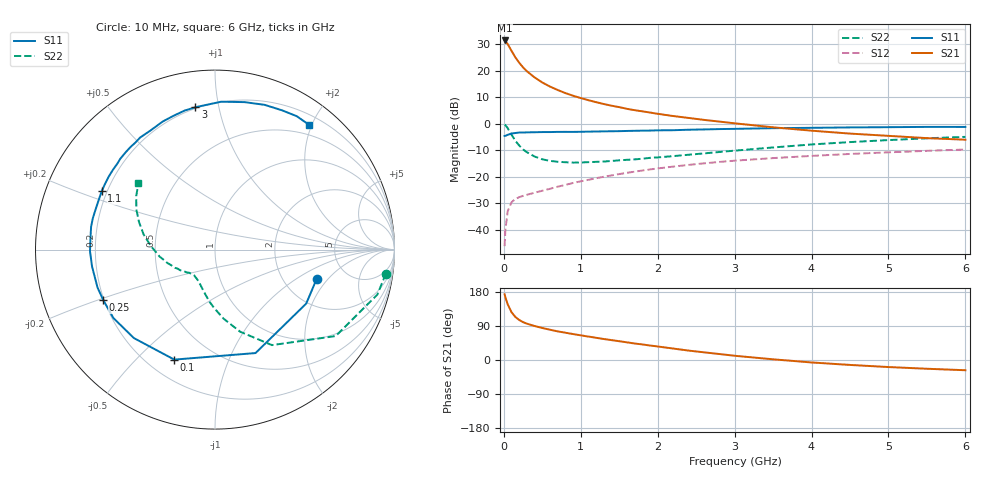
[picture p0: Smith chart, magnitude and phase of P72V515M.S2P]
! SIEMENS Small Signal Semiconductors
! BFP196
! Si NPN RF Bipolar Junction Transistor in SOT143
! VCE = 2.5 V  IC = 15 mA
! Common Emitter S-Parameters:  May  1996
# GHz  S  MA  R  50
!  f  S11  S21  S12  S22
! GHz  MAG  ANG  MAG  ANG  MAG  ANG  MAG  ANG
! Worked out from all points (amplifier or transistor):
!   36 points, 10 MHz to 6 GHz, reference 50 ohm
!   highest |S21| = 31.4 dB at 10 MHz (marker M1)
!   |S21| within 3 dB of that: start of sweep to 82.1 MHz
!   unconditionally stable (mu >= 1): 753.9 MHz to 3.377 GHz
!   at 250 MHz: K = 0.52, MSG = 24.2 dB, |S12| = -27.2 dB
!   at 1.4 GHz: K = 1.13, MAG = 11.0 dB, |S12| = -19.5 dB
!   at 6 GHz: K = 0.97, MSG = 1.9 dB, |S12| = -9.7 dB
!   S11 on the Smith chart (normalised r, x): 10 MHz: 3.06, -1.51; 100 MHz: 0.30, -0.65; 250 MHz: 0.20, -0.21; 1.1 GHz: 0.18, +0.23; 3 GHz: 0.19, +0.85; 6 GHz: 0.34, +1.96
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0.01  0.5897 -15.9  37.27 173.4  0.0049 84.6  0.9616 -8.0
0.02  0.5906 -30.6  35.82 165.3  0.0099 75.6  0.9386 -15.5
0.05  0.6191 -68.6  31.86 147.0  0.0223 62.6  0.8272 -35.6
0.1  0.6535 -110.3  23.75 126.0  0.033 47.8  0.6196 -59.2
0.15  0.6687 -132.5  17.85 113.5  0.0383 40.2  0.4781 -73.0
0.2  0.6825 -146.0  14.16 105.6  0.0412 37.8  0.3879 -82.9
0.25  0.6832 -155.7  11.55 99.9  0.0436 37.0  0.327 -90.6
0.3  0.6878 -162.1  9.785 95.9  0.0457 38.1  0.2905 -96.3
0.4  0.6914 -172.1  7.478 89.7  0.05 39.5  0.2405 -105.3
0.5  0.6965 -179.2  6.005 84.5  0.0545 41.9  0.2133 -112.3
0.6  0.6967 174.8  5.027 79.9  0.0592 43.8  0.1994 -117.6
0.7  0.7021 169.5  4.334 75.5  0.0649 45.5  0.1917 -121.9
0.8  0.7027 165.4  3.79 72.0  0.0702 46.6  0.1878 -125.5
1.1  0.7099 152.8  2.781 61.8  0.0876 49.0  0.1886 -133.8
1.3  0.7183 145.5  2.354 55.4  0.1001 49.0  0.1936 -138.3
1.6  0.7313 136.1  1.913 46.6  0.1186 47.9  0.2087 -144.1
2.2  0.7548 118.3  1.398 30.3  0.1553 43.3  0.2451 -155.6
3  0.8007 97.8  1.019 11.2  0.201 34.6  0.3107 -172.7
3.5  0.8247 87.6  0.857 1.8  0.2249 28.8  0.3569 177.0
4.5  0.8526 71.1  0.652 -13.0  0.2694 17.5  0.4507 160.0
5.5  0.8718 58.5  0.535 -23.1  0.3084 6.6  0.5311 145.7
6  0.8707 53.0  0.5 -27.0  0.3264 0.7  0.5656 138.9
